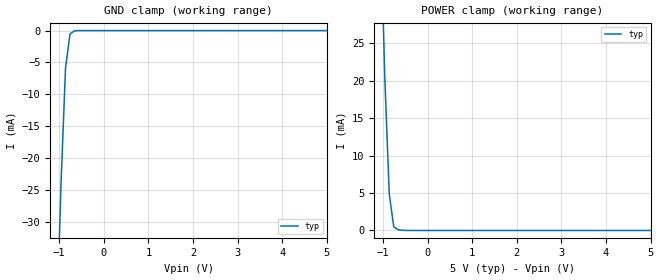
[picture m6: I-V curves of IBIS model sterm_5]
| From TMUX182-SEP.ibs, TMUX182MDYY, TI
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| sterm_5
[Model]   sterm_5
Model_type   Terminator
|   typ   min   max
C_comp   4.014581e-12   NA   NA
[Voltage Range]   5   NA   NA
[Temperature Range]   27   NA   NA
[Power Clamp Reference]   5   NA   NA
[GND Clamp Reference]   0   NA   NA
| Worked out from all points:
|   GND clamp passes 1 mA (typ) near -0.77 V on its own axis
|   POWER clamp passes 1 mA (typ) near -0.77 V on its own axis
[GND Clamp]
|   Voltage   I(typ)   I(min)   I(max)
-5V       -2.321A    NA         NA
-1.061V   -47.66mA   NA         NA
-959.6mV  -24.14mA   NA         NA
-858.6mV  -5.886mA   NA         NA
-757.6mV  -521uA     NA         NA
-656.6mV  -31.63uA   NA         NA
5V        53.43pA    NA         NA
[POWER Clamp]
|   Voltage   I(typ)   I(min)   I(max)
-5V       1.914A     NA         NA
-1.061V   43.19mA    NA         NA
-959.6mV  20.55mA    NA         NA
-858.6mV  4.892mA    NA         NA
-757.6mV  467.7uA    NA         NA
-656.6mV  105.7uA    NA         NA
-454.6mV  1.681uA    NA         NA
5V        -29.79pA   NA         NA
